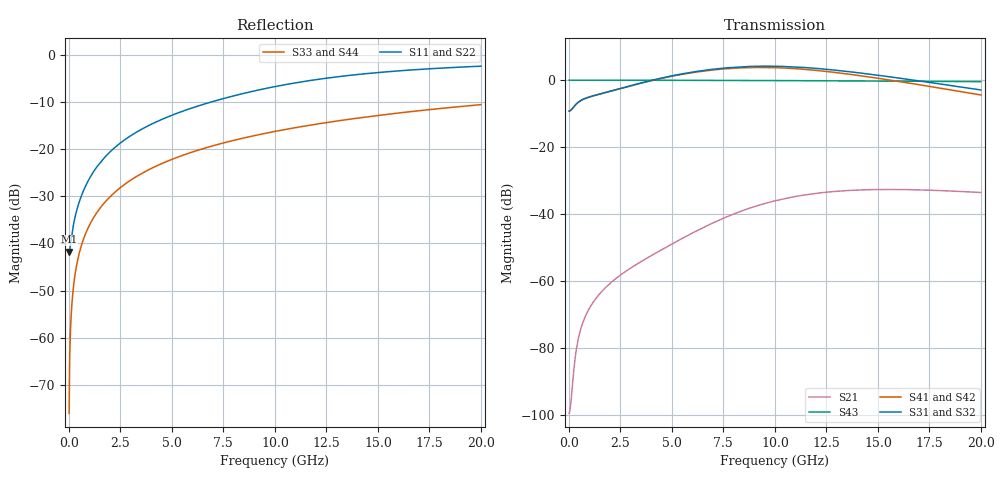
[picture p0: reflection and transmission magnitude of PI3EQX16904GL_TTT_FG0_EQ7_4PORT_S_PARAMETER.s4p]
! NPort=4 DATA=2000 NOISE=0 GROUPDELAY=0 COMPLEX_DATAFORMAT=POLAR
! NumOfBlock=1 NumOfParam=0
! .MODEL Smodel S TSTONEFILE=PI3EQX16904GL_TTT_FG0_EQ7_4PORT_S_PARAMETER.s4p TYPE=S
!  -- The above .MODEL line can be used for the S element in the netlist.
! The s parameter is extracted from the linear redriver, it is not bi-directional; only s(4,1)s(4,2) and s(3,1)s(3,2)
! should be the insertion loss
!Port definition:
!Port1 = input+
!Port2 = input-
!Port3 = output+
!Port4 = output-
# Hz S MA R  50
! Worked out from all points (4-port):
!   2000 points, 10 MHz to 20 GHz, reference 50 ohm
!   strongest paths, dB at 10 MHz, 5.01 GHz, 10.01 GHz, 15.01 GHz, 20 GHz:
!     S31: -9.2, 1.3, 4.2, 1.5, -2.9
!     S32: -9.2, 1.3, 4.1, 1.3, -3.1
!     S41: -9.2, 1.2, 3.7, 0.6, -4.4
!     S42: -9.2, 1.2, 3.7, 0.4, -4.6
!     S43: 0.0, 0.0, -0.1, -0.3, -0.4
!     S21: -99.6, -48.9, -36.1, -32.7, -33.6
!   lowest |S11| = -41.7 dB at 10 MHz (marker M1), VSWR 1.02, Z = 49.2 - j0.0603 ohm
!   |S11| at or under -10 dB: start of sweep to 6.858 GHz
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1e7  0.008182 -175.7  1.05e-05 7.8  0 0.0  0 0.0
     1.05e-05 7.8  0.008182 -175.7  0 0.0  0 0.0
     0.3452 0.7  0.3452 -179.3  0.0001571 -90.0  1 -0.0
     0.3452 -179.3  0.3452 0.7  1 -0.0  0.0001571 -90.0
3.8e8  0.02256 -119.7  0.0001026 118.5  0 0.0  0 0.0
       0.0001026 118.5  0.02256 -119.7  0 0.0  0 0.0
       0.4471 15.4  0.4472 -164.7  0.005969 -90.4  1 -0.3
       0.4471 -165.3  0.4472 14.7  1 -0.3  0.005969 -90.4
1.56e9  0.07424 -102.9  0.0006764 110.7  0 0.0  0 0.0
        0.000676 110.7  0.07423 -102.9  0 0.0  0 0.0
        0.6284 10.1  0.6294 -170.0  0.0245 -91.5  0.9997 -1.4
        0.6276 -172.7  0.6286 7.2  0.9997 -1.4  0.0245 -91.5
5.76e9  0.2652 -104.2  0.004798 109.4  0 0.0  0 0.0
        0.004761 109.8  0.2652 -104.2  0 0.0  0 0.0
        1.285 -33.6  1.28 145.7  0.09008 -95.4  0.9956 -5.2
        1.264 136.2  1.259 -44.5  0.9956 -5.2  0.09008 -95.4
9.37e9  0.4348 -111.1  0.01405 75.7  0 0.0  0 0.0
        0.01395 76.7  0.4347 -111.1  0 0.0  0 0.0
        1.619 -95.1  1.605 84.1  0.1455 -98.7  0.9885 -8.4
        1.551 68.5  1.538 -112.3  0.9885 -8.4  0.1455 -98.7
1.336e10  0.6014 -121.7  0.02235 24.2  0 0.0  0 0.0
          0.02225 25.7  0.6015 -121.7  0 0.0  0 0.0
          1.367 -162.2  1.348 16.8  0.205 -102.3  0.977 -11.8
          1.256 -4.9  1.24 174.1  0.977 -11.8  0.205 -102.3
2e10  0.7648 -136.6  0.02097 -38.2  0 0.0  0 0.0
      0.021 -35.9  0.7654 -136.6  0 0.0  0 0.0
      0.7143 111.0  0.6981 -70.1  0.2986 -108.1  0.9506 -17.4
      0.6015 -101.0  0.5878 78.0  0.9506 -17.4  0.2986 -108.1
